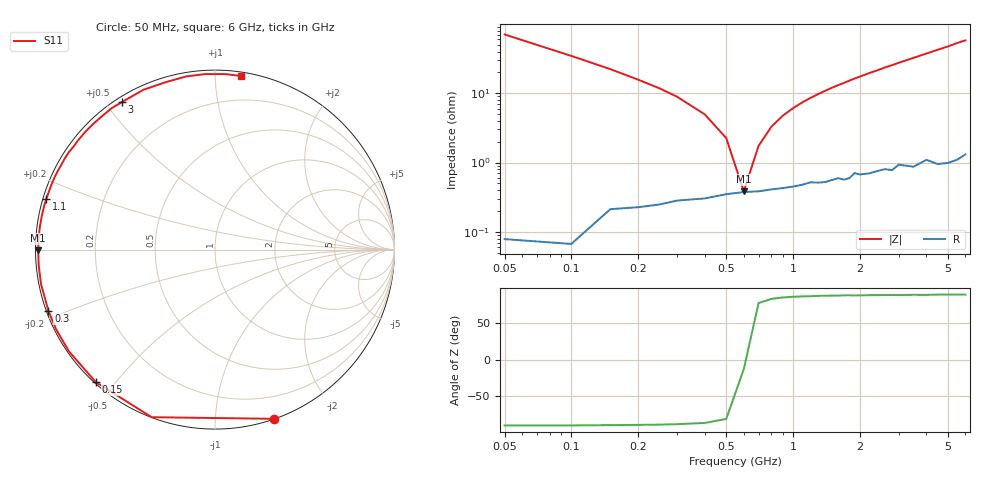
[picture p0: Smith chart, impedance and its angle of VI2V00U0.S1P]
! Infineon Technologies  Discrete & RF Semiconductors
! BB 804
! Si Tuning Diode in SOT23
! VR = 2 V
! S-Parameters:  July  1999
# GHz  S  MA  R  50
!  f  S11
! GHz  MAG  ANG
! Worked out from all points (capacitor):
!   34 points, 50 MHz to 6 GHz, reference 50 ohm
!   read as one part to ground: C = 44.8 pF near 50 MHz
!   lowest |Z| = 385 mohm at 600 MHz (marker M1)
!   series resonance near 604.9 MHz, so ESL is about 1.5 nH
!   S11 on the Smith chart (normalised r, x): 50 MHz: 0.00, -1.41; 150 MHz: 0.00, -0.45; 300 MHz: 0.01, -0.18; 1.1 GHz: 0.01, +0.15; 3 GHz: 0.02, +0.55; 6 GHz: 0.03, +1.16
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0.05  0.999 -70.7
0.1  0.9982 -110.7
0.15  0.9929 -132.0
0.2  0.9918 -145.1
0.25  0.9906 -153.5
0.3  0.9891 -159.8
0.4  0.988 -168.7
0.5  0.9861 -174.9
0.6  0.9851 -179.8
0.7  0.9848 176.1
0.8  0.9838 172.5
0.9  0.9832 169.2
1.1  0.9815 163.3
1.3  0.9804 158.0
1.6  0.978 150.7
1.7  0.9792 148.5
1.9  0.9748 143.8
2.2  0.9761 137.5
2.4  0.9748 133.7
2.6  0.974 129.6
2.8  0.9757 126.1
3  0.9718 122.4
3.5  0.9758 114.1
4  0.9723 106.4
4.5  0.9781 99.4
5  0.9794 93.2
5.5  0.9795 86.7
6  0.9779 81.6
